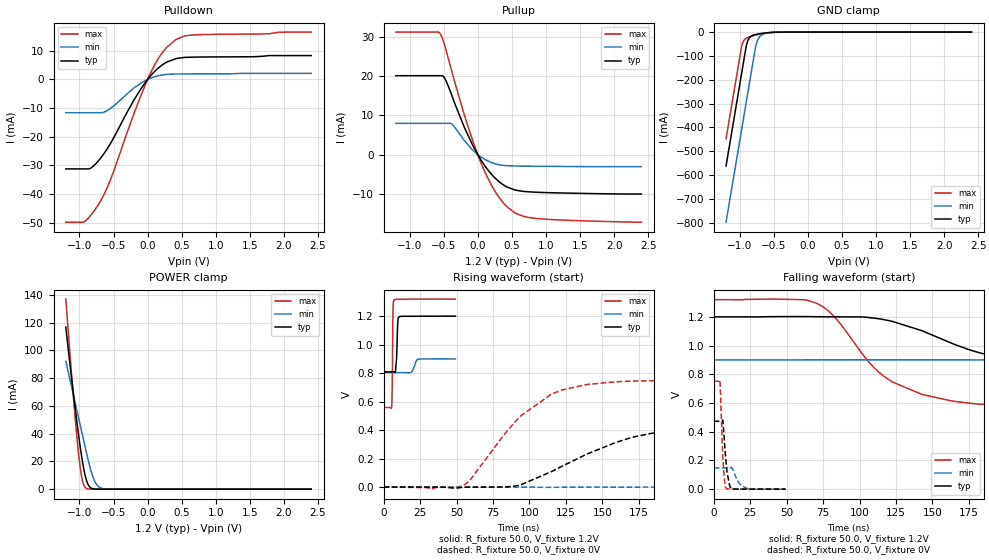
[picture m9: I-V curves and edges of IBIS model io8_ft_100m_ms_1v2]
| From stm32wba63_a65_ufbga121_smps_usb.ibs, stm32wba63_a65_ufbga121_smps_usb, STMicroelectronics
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[Model]   io8_ft_100m_ms_1v2
Model_type I/O
Polarity   Non-Inverting
Enable   Active-Low
| CAP_THRESHOLD on pad IOFT is "UDTCAPC" :
| Rising=30.0% of vddiom   Falling=70.0% of vddiom
| C_comp min and max val. don't necessarily correlate with the min and max pvt
| but are the smallest and greatest pad capacitance found.
| var   typ   min   max
C_comp   2.87220pF  2.79491pF  2.97971pF
|C_comp_pullup   1.64312pF  1.48357pF  1.78452pF
|C_comp_pulldown   1.22907pF  1.31134pF  1.19519pF
Vinl = 450.0mV
Vinh = 660.0mV
Vmeas = 600.0mV   | Reference voltage for timing measurements
Cref  = 50.0pF   | Timing specification test load capacitance value
Rref  = 1.0MOhm   | Timing specification test load resistance value
Vref  = 660.0mV   | Timing specification test load voltage
[Model Spec]
| TIME_THRESHOLD on pin ZIV11 is "CMOS" :
| Rising=50.0% of vdd   Falling=50.0% of vdd
Vinl 441.50000mV 335.50000mV 487.50000mV
Vinh 755.50000mV 552.50000mV 839.50000mV
| variable   typ   min   max
[Temperature Range] 25.0 140.0 -40.0
| variable   typ   min   max
[Voltage Range] 1.2V 900.0mV 1.32V
| variable   typ   min   max
[POWER Clamp Reference] 1.2V 900.0mV 1.32V
| variable   typ   min   max
[GND Clamp Reference] 0V 0V 0V
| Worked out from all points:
|   slope of the pulldown table from 0 to 0.18 V, typ, clamps not added: 40.6 ohm
|   slope of the pullup table from 0 to 0.18 V, typ, clamps not added: 39.4 ohm
|   GND clamp passes 1 mA (typ) near -0.51 V on its own axis
|   POWER clamp passes 1 mA (typ) near -0.83 V on its own axis
|   rising waveform, R_fixture 50.0, V_fixture 1.2V: 20-80 % time 786ps typ, 2.02ns min, 412ps max; typ from 0.809 V to 1.2 V
|   falling waveform, R_fixture 50.0, V_fixture 1.2V: 20-80 % time 79.8ns typ, 183ns min, 45.4ns max; typ from 1.2 V to 0.809 V
|   rising waveform, R_fixture 50.0, V_fixture 0V: 20-80 % time 72.5ns typ, 173ns min, 41.3ns max; typ from 0 V to 0.473 V
|   falling waveform, R_fixture 50.0, V_fixture 0V: 20-80 % time 2.55ns typ, 4.8ns min, 1.84ns max; typ from 0.473 V to 0 V
[POWER Clamp]
-1.2V     116.7mA    92.13mA    136.9mA
-1.09V    69.42mA    68.21mA    67.14mA
-1.02V    41.75mA    52.99mA    28.91mA
-990mV    30.98mA    46.47mA    16.09mA
-970mV    24.36mA    42.12mA    9.575mA
-940mV    15.59mA    35.6mA     3.485mA
-910mV    8.693mA    29.07mA    1.01mA
-860mV    2.259mA    18.59mA    104.6uA
-780mV    143.1uA    6.246mA    2.555uA
-720mV    16.22uA    1.846mA    157.1nA
-650mV    1.267uA    330.3uA    6.118nA
2.4V      0A         0A         0A
[GND Clamp]
-1.2V     -561.6mA   -797.4mA   -447.4mA
-980mV    -187.6mA   -423.4mA   -73.43mA
-960mV    -153.6mA   -389.4mA   -48.26mA
-900mV    -54.17mA   -287.4mA   -24.97mA
-870mV    -29.55mA   -236.4mA   -21.19mA
-830mV    -17.05mA   -168.4mA   -17.42mA
-760mV    -9.921mA   -54.55mA   -11.89mA
-730mV    -8.191mA   -29.78mA   -9.811mA
-690mV    -6.26mA    -14.49mA   -7.318mA
-600mV    -2.976mA   -4.315mA   -3.058mA
-380mV    -57.63uA   -251uA     -19.49uA
2.4V      872.8pA    204.8nA    349.4pA
| variable   typ   min   max
[Pullup Reference] 1.2V 900.0mV 1.32V
| variable   typ   min   max
[Pulldown Reference] 0V 0V 0V
[Pullup]
-1.2V     20.06mA    7.936mA    31.15mA
-580mV    20.06mA    7.936mA    31.15mA
-550mV    20.06mA    7.936mA    30.73mA
-480mV    19.26mA    7.936mA    27.49mA
-380mV    15.01mA    7.756mA    21.16mA
-200mV    7.069mA    3.64mA     10.26mA
20mV      -590.5uA   -260.8uA   -901.4uA
230mV     -5.55mA    -2.199mA   -8.66mA
440mV     -8.335mA   -2.843mA   -13.44mA
570mV     -9.105mA   -2.921mA   -15.05mA
790mV     -9.528mA   -2.972mA   -16.12mA
2.4V      -10.04mA   -3.075mA   -17.21mA
[Pulldown]
-1.2V     -31.2mA    -11.62mA   -49.78mA
-930mV    -31.2mA    -11.62mA   -49.64mA
-830mV    -30.86mA   -11.62mA   -47.25mA
-710mV    -28.04mA   -11.62mA   -43.19mA
-550mV    -22.55mA   -10.2mA    -35.3mA
-200mV    -7.146mA   -2.964mA   -11.89mA
40mV      1.171mA    405.8uA    2.092mA
130mV     3.416mA    1.118mA    6.182mA
230mV     5.302mA    1.613mA    9.763mA
420mV     7.288mA    1.898mA    13.99mA
670mV     7.779mA    1.924mA    15.51mA
2.4V      8.312mA    2.101mA    16.51mA
[Ramp]
dV/dt_r 283.79486mV/13.91318ns 88.93483mV/33.9664ns 450.99282mV/7.80918ns
dV/dt_f 234.65981mV/15.12407ns 57.89558mV/36.0154ns 456.73593mV/8.71277ns
R_load = 50.0
| Removed startup time: 0s 0s 0s  .
| Removed end time: 49.25ns.
[Rising Waveform]
R_fixture   = 50.0
V_fixture   = 1.2V
V_fixture_min = 900.0mV
V_fixture_max = 1.32V
0s        808.9mV    803.5mV    558.8mV
5.45ns    808.9mV    803.5mV    560.4mV
5.9ns     808.9mV    803.5mV    722.4mV
6.4ns     809mV      803.5mV    1.239V
7.05ns    808.5mV    803.5mV    1.313V
8.85ns    900mV      803.5mV    1.318V
10.05ns   1.188V     803.5mV    1.319V
19.1ns    1.199V     806.8mV    1.32V
23.15ns   1.199V     895.8mV    1.32V
49.25ns   1.2V       899.7mV    1.32V
| Removed startup time: 0s 0s 0s  .
| Removed end time: 1.99625us.
[Falling Waveform]
R_fixture   = 50.0
V_fixture   = 1.2V
V_fixture_min = 900.0mV
V_fixture_max = 1.32V
0s        1.2V       900mV      1.32V
69.5ns    1.201V     900.6mV    1.299V
81.75ns   1.2V       900.6mV    1.21V
106.8ns   1.195V     900.4mV    881.3mV
122.2ns   1.169V     900.5mV    747.8mV
163ns     1.017V     900.3mV    614.9mV
203.8ns   902.6mV    900mV      577.5mV
285.3ns   831.8mV    895.4mV    561.2mV
407.5ns   811.9mV    849.8mV    558.9mV
1.996us   808.9mV    803.5mV    558.8mV
| Removed startup time: 0s 0s 0s  .
| Removed end time: 1.996us.
[Rising Waveform]
R_fixture   = 50.0
V_fixture   = 0V
V_fixture_min = 0V
V_fixture_max = 0V
0s        4.648nV    215.3nV    3.229nV
53.75ns   -2.33mV    543.6nV    8.354mV
59.5ns    -601.7uV   182nV      52.07mV
92ns      10.79mV    -266.6uV   478.1mV
115.3ns   109.3mV    -2.067mV   653.6mV
168.5ns   343.3mV    -35.91uV   743.2mV
203.8ns   418.3mV    172.5uV    749.7mV
311ns     469.4mV    35.54mV    751.5mV
611ns     472.9mV    141.4mV    751.6mV
1.996us   473mV      148.2mV    751.7mV
| Removed startup time: 0s 0s 0s  .
| Removed end time: 49.25ns.
[Falling Waveform]
R_fixture   = 50.0
V_fixture   = 0V
V_fixture_min = 0V
V_fixture_max = 0V
0s        473mV      148.3mV    751.7mV
4.2ns     473mV      148.3mV    755mV
6.25ns    475.3mV    148.3mV    216.5mV
7.45ns    313.4mV    148.3mV    54.51mV
8.05ns    231.4mV    148.3mV    10.98mV
9.1ns     118.9mV    148.3mV    2.707mV
12.05ns   3.101mV    151.8mV    1.043mV
17.65ns   509.2uV    38.05mV    476.3uV
22.15ns   427.1uV    8.186mV    215.3uV
49.25ns   46.9uV     92.62uV    5.772uV
